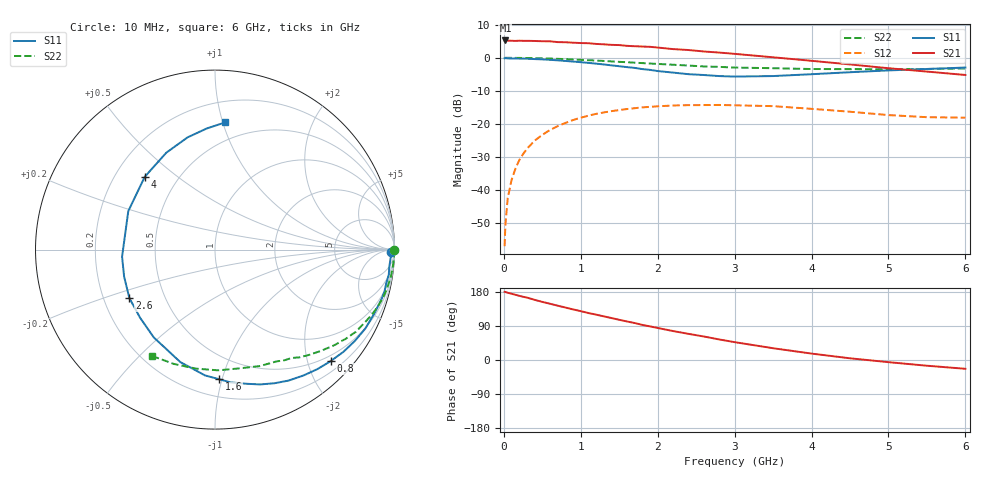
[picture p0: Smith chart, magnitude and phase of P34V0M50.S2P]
! SIEMENS Small Signal Semiconductors
! BFP181
! Si NPN RF Bipolar Junction Transistor in SOT143
! VCE = 4 V  IC = 0.5 mA
! Common Emitter S-Parameters:  March  1996
# GHz  S  MA  R  50
!  f  S11  S21  S12  S22
! GHz  MAG  ANG  MAG  ANG  MAG  ANG  MAG  ANG
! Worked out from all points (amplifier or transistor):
!   36 points, 10 MHz to 6 GHz, reference 50 ohm
!   highest |S21| = 5.2 dB at 20 MHz (marker M1)
!   |S21| within 3 dB of that: start of sweep to 2.447 GHz
!   unconditionally stable (mu >= 1): 3.769 GHz to end of sweep
!   at 250 MHz: K = 0.07, MSG = 17.2 dB, |S12| = -29.2 dB
!   at 1.4 GHz: K = 0.43, MSG = 10.0 dB, |S12| = -16.2 dB
!   at 6 GHz: K = 1.45, MAG = 2.5 dB, |S12| = -18.1 dB
!   S11 on the Smith chart (normalised r, x): 10 MHz: 68, -49; 800 MHz: 0.39, -2.43; 1.6 GHz: 0.32, -0.98; 2.6 GHz: 0.31, -0.24; 4 GHz: 0.32, +0.39; 6 GHz: 0.36, +1.02
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0.01  0.9807 -0.8  1.828 179.8  0.0014 72.0  0.9992 -0.2
0.02  0.9887 -1.4  1.83 179.5  0.0029 90.5  0.9977 -0.6
0.05  0.9797 -2.6  1.818 177.5  0.0074 91.6  0.9988 -1.3
0.1  0.976 -5.6  1.811 174.8  0.014 86.1  0.9979 -2.7
0.15  0.9784 -8.3  1.8 172.2  0.0208 83.4  0.9965 -4.0
0.2  0.9724 -11.0  1.814 169.4  0.0281 82.1  0.9956 -5.3
0.3  0.968 -16.6  1.807 164.8  0.0418 78.1  0.9923 -8.0
0.4  0.9556 -22.1  1.797 158.8  0.0554 74.7  0.9872 -10.6
0.6  0.9306 -33.2  1.775 148.5  0.0805 66.5  0.9735 -15.9
0.8  0.8955 -43.9  1.719 138.5  0.103 58.8  0.9542 -20.7
1.1  0.8369 -60.7  1.661 123.9  0.1328 48.3  0.9193 -27.7
1.5  0.7449 -83.3  1.558 106.1  0.1615 35.5  0.8676 -36.1
1.6  0.7221 -88.3  1.516 101.7  0.1674 32.7  0.8572 -37.9
1.9  0.656 -107.1  1.465 88.7  0.1808 24.2  0.818 -43.5
2.2  0.5964 -124.9  1.354 76.4  0.1893 16.7  0.7848 -48.5
2.6  0.5482 -150.5  1.246 62.0  0.1921 7.9  0.7391 -54.8
3  0.5193 -175.6  1.147 47.1  0.1906 -0.6  0.7109 -61.2
3.5  0.5285 156.1  1.017 31.1  0.1851 -8.7  0.6952 -69.0
4  0.5636 134.0  0.9 16.9  0.1685 -14.8  0.6757 -78.3
4.5  0.6042 116.7  0.793 4.5  0.1524 -19.3  0.6729 -88.5
5.5  0.6764 93.9  0.618 -15.1  0.1259 -15.7  0.6771 -109.8
6  0.7115 85.3  0.549 -23.2  0.1238 -11.6  0.6889 -120.9
